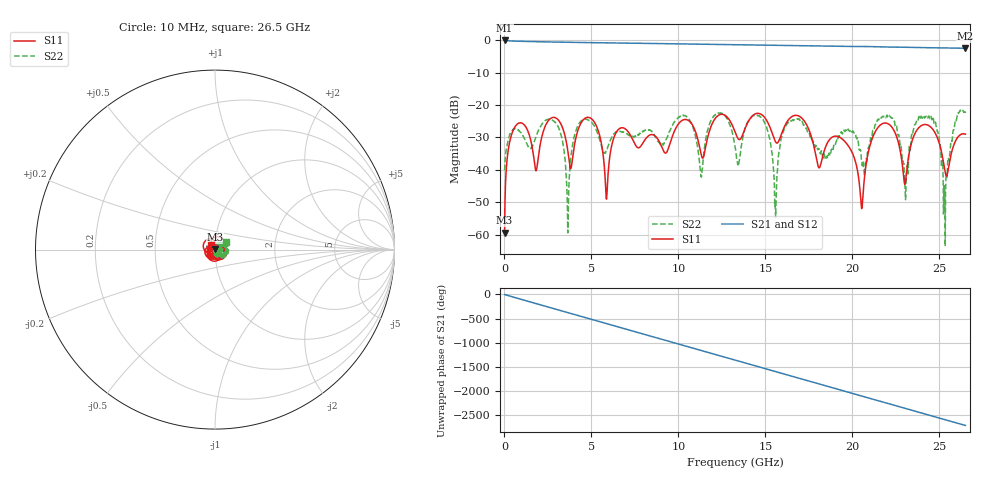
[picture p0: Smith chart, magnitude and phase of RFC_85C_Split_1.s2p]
!Keysight Technologies,N5245B,MY55451909,A.13.80.08
!Automatic Fixture Removal (AFR)
!Date: Thursday, August 27, 2020, 03:53:37
!S2P File: Measurements: S11,S21,S12,S22:
# MHz S  RI  R 50
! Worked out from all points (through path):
!   2650 points, 10 MHz to 26.5 GHz, reference 50 ohm
!   highest |S21| = -0.01 dB at 10 MHz (marker M1); lowest = -2.4 dB at 26.48 GHz (marker M2)
!   group delay of S21, straight-line fit = 285 ps
!   lowest |S11| = -59.4 dB at 10 MHz (marker M3), VSWR 1.00, Z = 50 + j0.107 ohm
!   |S11| at or under -10 dB: start of sweep to end of sweep
!   |S22| runs from -63.6 to -21.3 dB; largest |S21 - S12| = 1.5e-15
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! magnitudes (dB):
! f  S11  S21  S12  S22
! 10 MHz  -59.4  0.0  0.0  -40.2
! 690 MHz  -26.1  -0.2  -0.2  -27.4
! 1.82 GHz  -40.3  -0.4  -0.4  -29.6
! 2.94 GHz  -23.9  -0.5  -0.5  -25.4
! 3.64 GHz  -34.0  -0.6  -0.6  -59.4
! 4.43 GHz  -25.3  -0.6  -0.6  -24.8
! 5.87 GHz  -49.1  -0.7  -0.7  -34.0
! 6.59 GHz  -27.3  -0.8  -0.8  -28.2
! 8.84 GHz  -30.7  -1.0  -1.0  -31.3
! 13.26 GHz  -28.3  -1.3  -1.3  -32.8
! 14.74 GHz  -22.8  -1.4  -1.4  -23.7
! 15.58 GHz  -31.3  -1.5  -1.5  -52.5
! 16.23 GHz  -25.3  -1.5  -1.5  -25.9
! 17.67 GHz  -30.2  -1.7  -1.7  -30.5
! 19.62 GHz  -31.5  -1.8  -1.8  -27.7
! 20.54 GHz  -52.0  -1.9  -1.9  -37.1
! 22.09 GHz  -25.9  -2.0  -2.0  -23.5
! 23.09 GHz  -42.2  -2.1  -2.1  -42.9
! 24.65 GHz  -27.6  -2.3  -2.3  -24.0
! 25.34 GHz  -40.8  -2.3  -2.3  -63.6
! 26.48 GHz  -28.9  -2.4  -2.4  -22.1
! 26.5 GHz  -29.0  -2.4  -2.4  -22.4
